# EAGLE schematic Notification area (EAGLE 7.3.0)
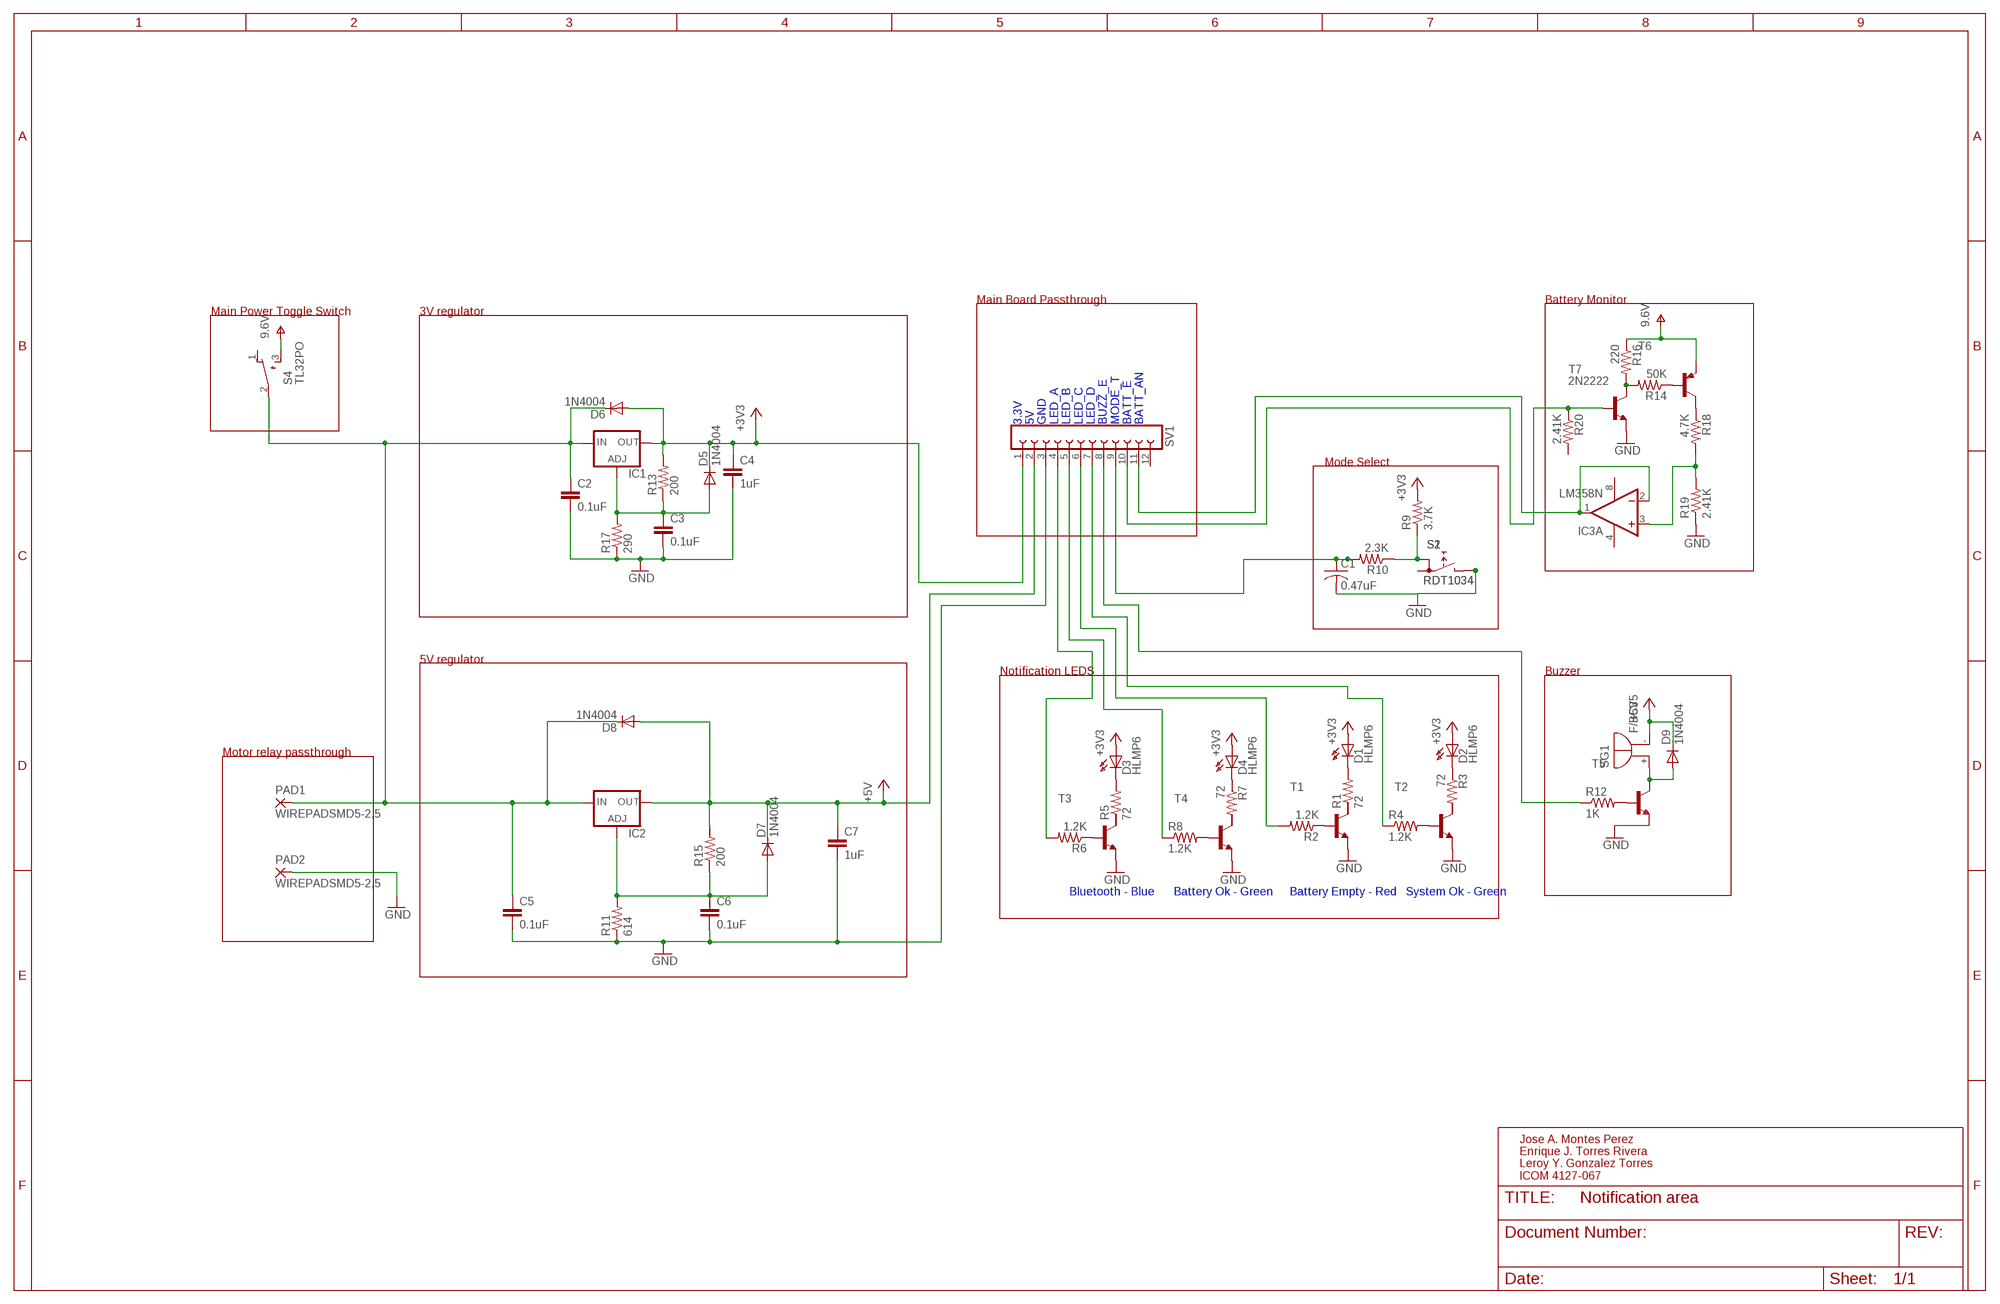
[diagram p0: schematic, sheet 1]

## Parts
C1  0.47uF  C-US025-030X050  [C025-030X050]
C2  0.1uF  C2,5-3  [C2.5-3]
C3  0.1uF  C2,5-3  [C2.5-3]
C4  1uF  C2,5-3  [C2.5-3]
C5  0.1uF  C2,5-3  [C2.5-3]
C6  0.1uF  C2,5-3  [C2.5-3]
C7  1uF  C2,5-3  [C2.5-3]
D1  HLMP6  [HLMP6]
D2  HLMP6  [HLMP6]
D3  HLMP6  [HLMP6]
D4  HLMP6  [HLMP6]
D5  1N4004  [DO41-10]
D6  1N4004  [DO41-10]
D7  1N4004  [DO41-10]
D8  1N4004  [DO41-10]
D9  1N4004  [DO41-10]
IC1  LM317TS  [317TS]
IC2  LM317TS  [317TS]
IC3  LM358N  [DIL08]
PAD1  WIREPADSMD5-2,5  [5-2,5]
PAD2  WIREPADSMD5-2,5  [5-2,5]
R1  72  R-US_0204/7  [0204/7]
R2  1.2K  R-US_0204/7  [0204/7]
R3  72  R-US_0204/7  [0204/7]
R4  1.2K  R-US_0204/7  [0204/7]
R5  72  R-US_0204/7  [0204/7]
R6  1.2K  R-US_0204/7  [0204/7]
R7  72  R-US_0204/7  [0204/7]
R8  1.2K  R-US_0204/7  [0204/7]
R9  3.7K  R-US_0204/7  [0204/7]
R10  2.3K  R-US_0204/7  [0204/7]
R11  614  R-US_0204/7  [0204/7]
R12  1K  R-US_0207/7  [0207/7]
R13  200  R-US_0204/7  [0204/7]
R14  50K  R-US_0204/7  [0204/7]
R15  200  R-US_0204/7  [0204/7]
R16  220  R-US_0204/7  [0204/7]
R17  290  R-US_0204/7  [0204/7]
R18  4.7K  R-US_0204/7  [0204/7]
R19  2.41K  R-US_0204/7  [0204/7]
R20  2.41K  R-US_0204/7  [0204/7]
S1  RDT1034  [RDT1034]
S2  RDT1034  [RDT1034]
S4  TL32PO  [TL3XPO]
SG1  F/BC35  [F/BC35]
SV1  FE12-1  [FE12]
T1  2N2222-NPN-TO92-EBC  [TO92-EBC]
T2  2N2222-NPN-TO92-EBC  [TO92-EBC]
T3  2N2222-NPN-TO92-EBC  [TO92-EBC]
T4  2N2222-NPN-TO92-EBC  [TO92-EBC]
T5  2N2222-NPN-TO92-EBC  [TO92-EBC]
T6  2N3906-PNP-TO92-EBC  [TO92-EBC]
T7  2N2222  [TO18]

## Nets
+3V3: C4.1 D1.A D2.A D3.A D4.A D5.C D6.A IC1.2(OUT) R9.2 R13.2 SV1.1
+5V: C7.1 D7.C D8.A D9.C IC2.2(OUT) R15.2 SG1.- SV1.2
GND: C1.2 C2.2 C3.2 C4.2 C5.2 C6.2 C7.2 PAD2.1(P) R11.1 R17.1 R19.1 SV1.3 T1.E T2.E T3.E T4.E T5.E T7.1(E)
N$1: D1.K R1.2
N$2: R2.1 T1.B
N$3: D2.K R3.1
N$4: R4.2 T2.B
N$5: D3.K R5.2
N$6: R6.1 T3.B
N$7: D4.K R7.1
N$8: R8.2 T4.B
N$9: R6.2 SV1.4
N$10: C1.1 R10.2 SV1.9
N$11: R8.1 SV1.5
N$12: R4.1 SV1.7
N$13: R9.1 R10.1 S1.A S2.A
N$14: C2.1 C5.1 D6.C D8.C IC1.3(IN) IC2.3(IN) PAD1.1(P) S4.2(P)
N$15: S1.B S2.B
N$16: R12.2 T5.B
N$17: S1.A1 S2.A1
N$18: R2.2 SV1.6
N$19: C3.1 D5.A IC1.1(ADJ) R13.1 R17.2
N$20: C6.1 D7.A IC2.1(ADJ) R11.2 R15.1
N$21: D9.A SG1.+ T5.C
N$22: R14.1 T6.B
N$23: R14.2 R16.2 T7.3(C)
N$24: R12.1 SV1.8
N$25: R18.1 T6.C
N$26: IC3.1(A:OUT) IC3.2(A:-IN) SV1.11
N$27: IC3.3(A:+IN) R18.2 R19.2
N$28: R20.1 SV1.10 T7.2(B)
V+: R16.1 S4.3(S) T6.E ; supply symbol labelled 9.6V
Unconnected: IC3.5(B:+IN) IC3.6(B:-IN) IC3.7(B:OUT) R1.1 R3.2 R5.1 R7.2 R20.2 S4.1(O) SV1.12 T1.C T2.C T3.C T4.C

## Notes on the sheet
- Main Board Passthrough | Battery Monitor
- Main Power Toggle Switch | 3V regulator
- 3.3V
  5V
  GND
  LED_A
  LED_B
  LED_C
  LED_D
  BUZZ_E
  MODE_T
  BATT_E
  BATT_AN
- Mode Select
- 5V regulator
- Notification LEDS | Buzzer
- Motor relay passthrough
- Bluetooth - Blue | Battery Ok - Green | Battery Empty - Red | System Ok - Green
- Jose A. Montes Perez
  Enrique J. Torres Rivera
  Leroy Y. Gonzalez Torres
  ICOM 4127-067

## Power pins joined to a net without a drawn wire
V+: IC3.8(P:V+)
V-: IC3.4(P:V-)

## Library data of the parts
C1 = rcl:C-US: CAPACITOR, American symbol
C2-C7 = capacitor-wima:C: CAPACITOR
D1-D4 = display-hp:HLMP6: LED; MF: AGILENT TECHNOLOGIES; MPN: HLMP-6500; OC_FARNELL: 1652490; OC_NEWARK: 40K0088
D5-D9 = diode:1N4004: DIODE
IC1 IC2 = v-reg:LM317TS: VOLTAGE REGULATOR
IC3 = linear:LM358: OP AMP also LM158; LM258; LM2904 Source: http://cache.national.com/ds/LM/LM158.pdf
PAD1 PAD2 = wirepad:WIREPAD: Wire PAD connect wire on PCB
R1-R20 = rcl:R-US_: RESISTOR, American symbol
S1 S2 = switch:RDT1034: PUSH SWITCH www.radiohm.com
S4 = switch:TL32PO: TINY SWITCH ON - MOM Source: http://www2.produktinfo.conrad.com/datenblaetter/700000-724999/705152-da-01-de-Subminiaturschalter_TL_36YO.pdf
SG1 = buzzer:F/BC35: BUZZER; OC_FARNELL: unknown; OC_NEWARK: unknown
SV1 = con-lsta:FE12-1: FEMALE HEADER; OC_FARNELL: unknown; OC_NEWARK: unknown
T1-T5 = transistor-neu-to92:*-NPN-: NPN Transistror
T6 = transistor-neu-to92:*-PNP-: PNP Transistror
T7 = transistor-neu-to92:2N2222: NPN TRANSISTOR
